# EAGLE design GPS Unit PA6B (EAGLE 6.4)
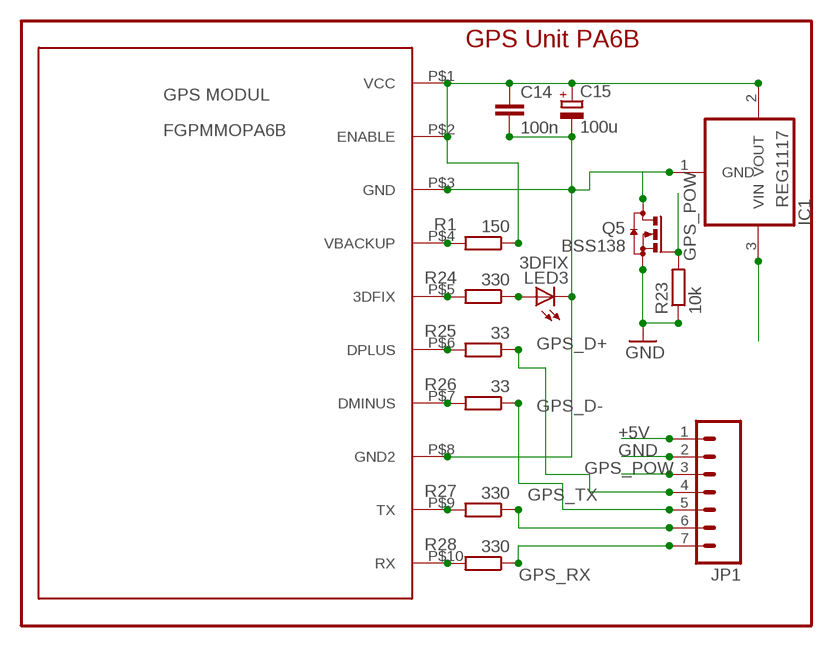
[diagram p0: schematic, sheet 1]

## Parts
C14  100n  C-EUC0805K  [C0805K]
C15  100u  CPOL-EUCT6032  [CT6032]
IC1  REG1117  [SOT223]
JP1  M07LOCK  [1X07_LOCK]
LED3  3DFIX  LEDSML0805  [SML0805]
PA6B1  MediaTek MT3329  GPS_MODUL_FGPMMOPA6B  [FGPMMOPA6B]
Q5  BSS138  BSS123  [SOT23]
R1  150  R-EU_M0805  [M0805]
R23  10k  R-EU_M0805  [M0805]
R24  330  R-EU_M0805  [M0805]
R25  33  R-EU_M0805  [M0805]
R26  33  R-EU_M0805  [M0805]
R27  330  R-EU_M0805  [M0805]
R28  330  R-EU_M0805  [M0805]

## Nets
3V3: C14.1 C15.+ IC1.2(VOUT) PA6B1.P$1(VCC) PA6B1.P$2(ENABLE) R1.1
+5V [power]: IC1.3(VIN) JP1.1
GND [power]: JP1.2 Q5.2(S) R23.1
GND_GPS: C14.2 C15.- IC1.1(GND) LED3.C PA6B1.P$3(GND) PA6B1.P$8(GND2) Q5.3(D)
GPS_D+: JP1.4 R25.1
GPS_D-: JP1.5 R26.1
GPS_POW [power]: JP1.3 Q5.1(G) R23.2
GPS_RX: JP1.7 R28.1
GPS_TX: JP1.6 R27.1
N$1: PA6B1.P$4(VBACKUP) R1.2
N$22: PA6B1.P$10(RX) R28.2
N$25: PA6B1.P$9(TX) R27.2
N$26: PA6B1.P$7(DMINUS) R26.2
N$30: PA6B1.P$6(DPLUS) R25.2
N$31: PA6B1.P$5(3DFIX) R24.2
N$55: LED3.A R24.1

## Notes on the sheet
- GPS Unit PA6B

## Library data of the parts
C14 = rcl:C-EU: CAPACITOR, European symbol
C15 = rcl:CPOL-EU: POLARIZED CAPACITOR, European symbol
IC1 = burr-brown:REG1117: 800mA and 1A Low Dropout (LDO) Positive Regulator 1.8V, 2.5V, 2.85V, 3.3V, 5V, and Adj; MPN: REG1117; OC_FARNELL: 1097566; OC_NEWARK: 14P6981
JP1 = SparkFun:M07: Header 7 Standard 7-pin 0.1" header. Use with straight break away headers (SKU : PRT-00116), right angle break away headers (PRT-00553), swiss pins (PRT-00743), machine pins (PRT-00117), and female headers (PRT-00115). NOTES ON THE VARIANTS LOCK and LOCK_LONGPADS... This footprint was designed to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
LED3 = led:LED: LED
PA6B1 = FGPMMOPA6B_GPS_MODUL:GPS_MODUL_FGPMMOPA6B
Q5 = transistor-small-signal:BSS123: N-CHANNEL MOS FET
R1 R23-R28 = resistor:R-EU_: RESISTOR, European symbol

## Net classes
0 default: width 0.254 mm, drill 0.406 mm, clearance 0.127 mm
1 power: width 0.305 mm, drill 0.813 mm, clearance 0.254 mm

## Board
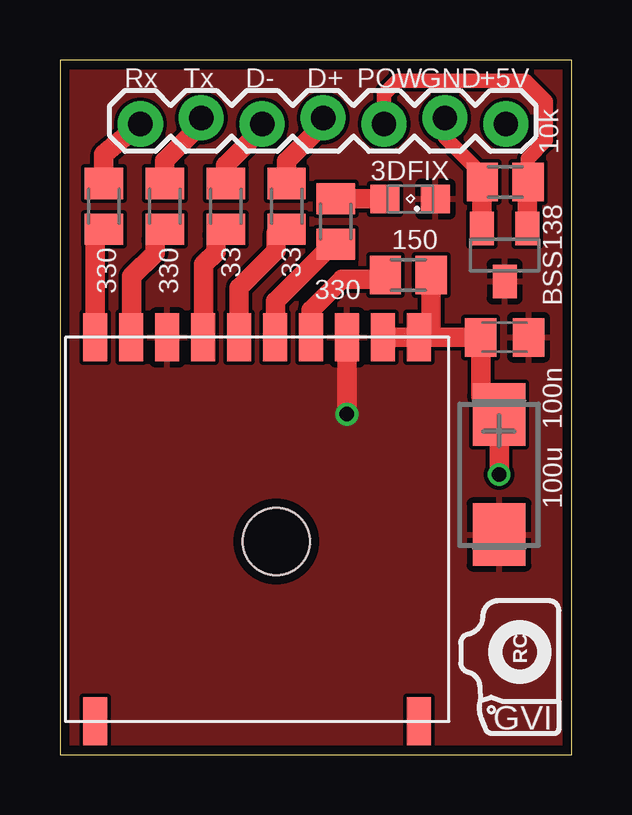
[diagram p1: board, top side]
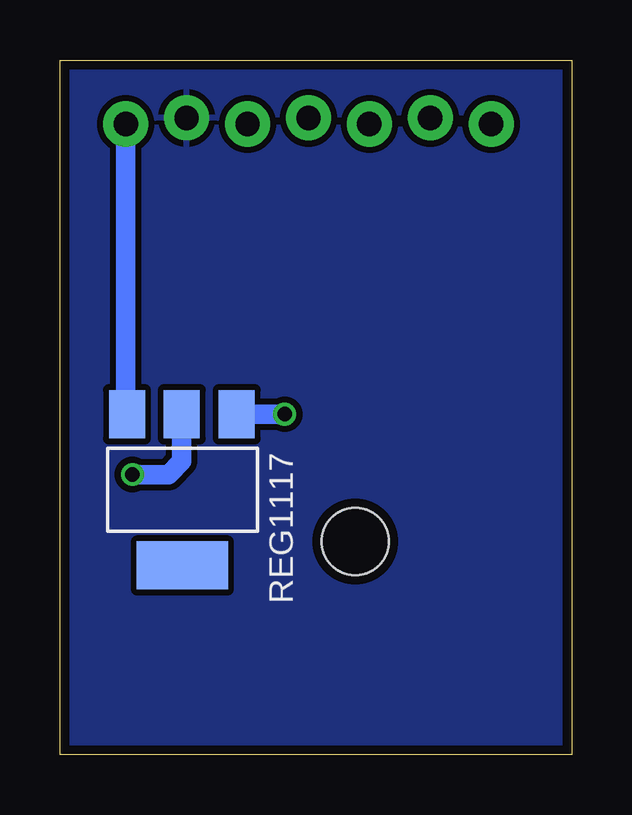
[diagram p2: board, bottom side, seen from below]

Size 21.34 x 28.96 mm. Coordinates in mm from the lower left corner, seen from the top.
Outline: 0,0 21.34,0 21.34,28.96 0,28.96 0,0
Copper layers (1*16): Top 0.0356mm / dielectric 1.5011mm / Bottom 0.0356mm
Design rules "LaenPCBOrder": minimum track width 6mil, minimum drill 13mil, track to track 6mil, track to pad 6mil, pad to pad 6mil, via to via 6mil, smd to smd 6mil, copper to edge 15mil, drill to drill 6mil, minimum pad ring 7mil, minimum via ring 7mil, stop-mask expansion 4mil, vias tented up to drill 0mil, thermal gap 10mil
Holes 2.8 mm at 9.02,8.89

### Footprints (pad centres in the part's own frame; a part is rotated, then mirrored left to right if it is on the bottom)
C0805K = smd 1.3 x 1.6: 1 -1,0; 2 1,0
CT6032 = smd 2.6 x 2.2: + -2.5,0; - 2.5,0
SOT223 = smd 1.499 x 2.007: 1 -2.261,-3.15; 2 0.025,-3.15; 3 2.311,-3.15 | smd 3.81 x 2.007: 4 0,3.15
1X07_LOCK = drill 1.016 pad 1.88: 1 0,0.127; 2 2.54,-0.127; 3 5.08,0.127; 4 7.62,-0.127; 5 10.16,0.127; 6 12.7,-0.127; 7 15.24,0.127
SML0805 = smd 1.2 x 1.2: A 1.05,0; C -1.05,0
FGPMMOPA6B = smd 2 x 1: P$1 0,14.75; P$2 0,13.25; P$3 0,11.75; P$4 0,10.25; P$5 0,8.75; P$6 0,7.25; P$7 0,5.75; P$8 0,4.25; P$9 0,2.75; P$10 0,1.25; P$11 16,14.75; P$12 16,1.25
SOT23 = smd 1 x 1.4: 1 -0.95,-1.1; 2 0.95,-1.1; 3 0,1.1
M0805 = smd 1.3 x 1.6: 1 -0.95,0; 2 0.95,0

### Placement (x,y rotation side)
C14  18.54,17.4 0 top
C15  18.31,11.68 270 top
IC1  16.23,11.05 180 bottom
JP1  18.59,26.42 180 top
LED3  14.61,23.16 180 top
PA6B1  0.23,17.4 270 top
Q5  18.54,20.83 180 top
R1  14.53,19.99 180 top
R23  18.57,23.88 0 top
R24  11.51,22.23 270 top
R25  9.45,22.86 270 top
R26  6.91,22.86 270 top
R27  4.37,22.86 270 top
R28  1.83,22.86 270 top
U$1  [LOGO-SS]  19.18,4.29 90 top

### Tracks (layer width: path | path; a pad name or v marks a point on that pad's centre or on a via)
3V3  (via drill 0.6)
  Top 0.813: 15.52,17.4 C14.1 17.54,14.96 C15.+ v18.31,11.68 | 15.52,17.4 PA6B1.P$1 PA6B1.P$2 | R1.1 15.48,17.44 15.52,17.4
  Bottom 0.813: IC1.2 16.26,12.24 16.82,11.68 v18.31,11.68
+5V
  Bottom 0.813: JP1.1 18.59,14.25 IC1.3
GND
  Top 0.61: R23.1 17.63,24.16 16.05,25.73 JP1.2
  Top 0.813: Q5.2 17.59,23.85 R23.1
  pour Bottom: 0,0 0,28.96 21.34,28.96 21.34,0
GND_GPS  (via drill 0.6)
  Top 0.813: v11.96,14.2 11.96,17.38 PA6B1.P$3
  Bottom 0.813: IC1.1 v11.96,14.2
  pour Top: 0,0 0,28.96 21.34,28.96 21.34,0
GPS_D+
  Top 0.813: R25.1 9.45,24.74 10.97,26.26 JP1.4
GPS_D-
  Top 0.813: R26.1 6.91,24.56 8.43,26.09 JP1.5
GPS_POW
  Top 0.61: R23.2 19.52,24.85 20.27,25.6 20.27,27.23 19.41,28.09 14.07,28.09 13.51,27.53 JP1.3
  Top 0.813: Q5.1 19.49,23.85 R23.2
GPS_RX
  Top 0.813: R28.1 1.83,25.02 JP1.7
GPS_TX
  Top 0.813: R27.1 4.37,24.77 5.89,26.29 JP1.6
N$1
  Top 0.813: PA6B1.P$4 10.48,18.53 11.76,19.81 13.4,19.81 R1.2
N$22
  Top 0.813: PA6B1.P$10 1.48,21.79 R28.2
N$25
  Top 0.813: R27.2 4.37,21.87 3.96,21.46 3.96,20.9 3,19.94 3,17.42 PA6B1.P$9
N$26
  Top 0.813: R26.2 6.91,22.07 6.5,21.67 6.5,20.95 5.99,20.45 5.99,17.41 PA6B1.P$7
N$30
  Top 0.813: PA6B1.P$6 7.48,19.47 9.02,21.01 9.02,21.73 R25.2
N$31
  Top 0.813: R24.2 11.37,21.27 8.99,18.9 8.99,17.41 PA6B1.P$5
N$55
  Top 0.813: R24.1 13.24,23.18 LED3.A

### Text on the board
tPlace: Rx | +5V | Tx | D- | D+ | POW | GND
